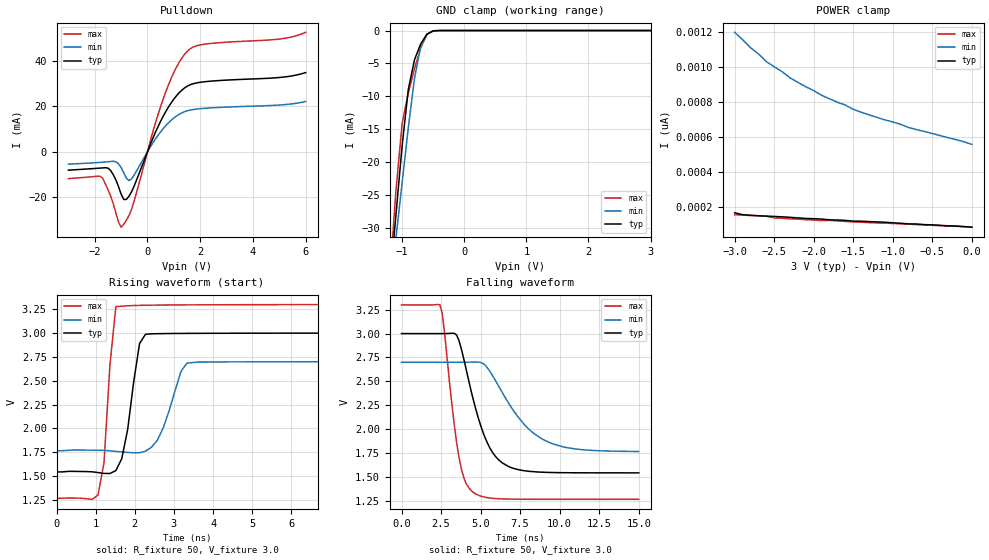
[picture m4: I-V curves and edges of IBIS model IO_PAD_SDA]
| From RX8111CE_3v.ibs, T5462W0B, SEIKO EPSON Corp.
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[Model]   IO_PAD_SDA
Model_type I/O_open_drain
Enable Active-High
Polarity Non-Inverting
Vinh=2.64
Vinl=0.54
Vmeas=1.50
Vref=3.3
Rref=5000
C_comp   2.5p   2.0p   3.0p
[Temperature Range] 25   105   -40
[Voltage Range]   3.0   2.7   3.3
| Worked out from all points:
|   slope of the pulldown table from 0 to 0.45 V, typ, clamps not added: 36.6 ohm
|   GND clamp passes 1 mA (typ) near -0.63 V on its own axis
|   falling waveform, R_fixture 50, V_fixture 3.0: 20-80 % time 1.52ns typ, 2.47ns min, 882ps max; typ from 3 V to 1.54 V
|   rising waveform, R_fixture 50, V_fixture 3.0: 20-80 % time 312ps typ, 452ps min, 203ps max; typ from 1.54 V to 3 V
[Pulldown]
-3V       -8.088mA   -5.43mA    -11.82mA
-1.7V     -7.087mA   -4.564mA   -11.64mA
-1.4V     -8.197mA   -4.255mA   -19.3mA
-1V       -18.62mA   -6.885mA   -33.2mA
-800mV    -20.97mA   -11.57mA   -30.12mA
-600mV    -17.54mA   -11.86mA   -25.25mA
600mV     15.77mA    10.27mA    23.45mA
1.1V      24.7mA     15.77mA    37.31mA
1.5V      28.87mA    18.05mA    44.2mA
2.1V      30.79mA    19.12mA    47.31mA
5V        32.75mA    20.62mA    49.7mA
6V        34.91mA    22.17mA    52.66mA
[GND Clamp]
-3V       -235.8mA   -196mA     -284.7mA
-1.2V     -38.9mA    -40.16mA   -37.89mA
-1.1V     -28.19mA   -31.69mA   -24.51mA
-1V       -17.59mA   -23.23mA   -14.19mA
-900mV    -8.97mA    -14.82mA   -9.504mA
-800mV    -4.445mA   -7.289mA   -5.814mA
-700mV    -2.032mA   -2.406mA   -2.637mA
-600mV    -545.2uA   -567.4uA   -605.7uA
-500mV    -56.87uA   -91.02uA   -35.51uA
3V        84.58pA    596.4pA    76.85pA
[POWER Clamp]
-3V       166.9pA    1.2nA      155.5pA
-2.9V     156pA      1.158nA    153.7pA
-2.8V     152.8pA    1.112nA    151pA
-2.7V     149.6pA    1.077nA    150.1pA
-2.6V     147.8pA    1.033nA    147.3pA
-2.5V     146pA      1.003nA    137.3pA
-2.3V     141pA      939.5pA    131.9pA
-1.9V     131pA      839.5pA    121.9pA
-1.5V     119.1pA    759.4pA    114.6pA
-1.3V     116.4pA    727.6pA    110.5pA
-800mV    103.2pA    655.3pA    101.9pA
0V        84.58pA    558.4pA    84.58pA
[Falling Waveform]
R_fixture=50
V_fixture=3.0
V_fixture_min=2.7
V_fixture_max=3.3
0s        3V         2.7V       3.3V
2.424ns   3V         2.7V       3.302V
2.576ns   3V         2.7V       3.213V
3.636ns   2.925V     2.7V       1.704V
4.091ns   2.623V     2.701V     1.43V
4.545ns   2.304V     2.702V     1.338V
5.606ns   1.797V     2.601V     1.279V
6.818ns   1.605V     2.26V      1.268V
9.545ns   1.547V     1.847V     1.266V
15ns      1.543V     1.767V     1.266V
[Rising Waveform]
R_fixture=50
V_fixture=3.0
V_fixture_min=2.7
V_fixture_max=3.3
0s        1.543V     1.765V     1.266V
1.061ns   1.536V     1.77V      1.301V
1.212ns   1.528V     1.769V     1.638V
1.364ns   1.526V     1.765V     2.661V
1.515ns   1.557V     1.759V     3.278V
1.818ns   1.991V     1.747V     3.286V
2.121ns   2.891V     1.744V     3.291V
2.273ns   2.988V     1.761V     3.292V
3.333ns   2.997V     2.685V     3.296V
15ns      3V         2.7V       3.3V
[Ramp]
R_load=50
dV/dt_r   8.743E-1/2.910E-10   5.608E-1/4.425E-10   1.220E+0/1.761E-10
dV/dt_f   8.743E-1/1.521E-9   5.600E-1/2.461E-9   1.220E+0/8.774E-10
|[End   IO_PAD_SDA
